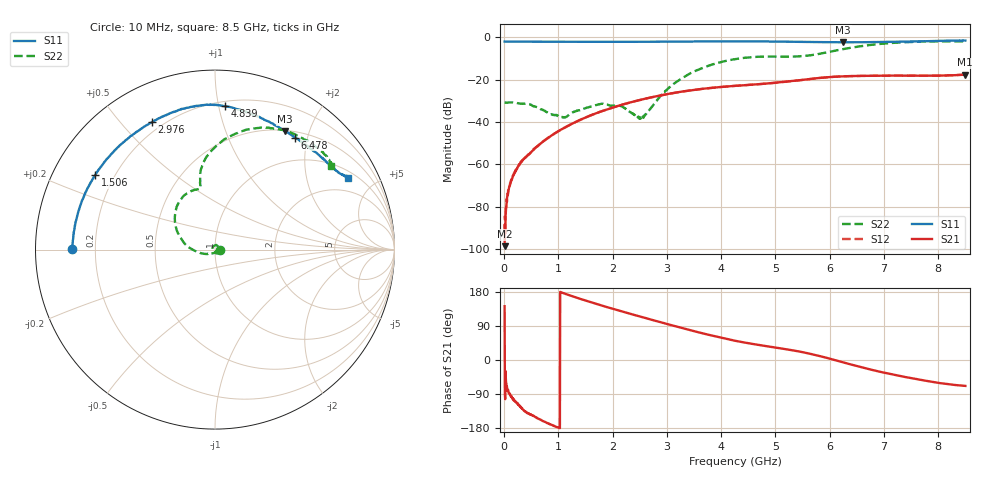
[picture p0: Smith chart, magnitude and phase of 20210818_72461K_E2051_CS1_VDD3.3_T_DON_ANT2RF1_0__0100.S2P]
!Agilent Technologies,E5071C,MY46417908,A.11.23
!Date: Wed Aug 18 14:23:03 2021
!Data & Calibration Information:
!Freq	S11:SOLT2(ON)	S21:SOLT2(ON)	S12:SOLT2(ON)	S22:SOLT2(ON)
!PortZ  Port1:50+j0  Port2:50+j0
!Above PortZ is port z conversion or system Z0 setting when saving the data.
!When reading, reference impedance value at option line is always used.
# Hz S dB R 50
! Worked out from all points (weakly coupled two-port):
!   1601 points, 10 MHz to 8.5 GHz, reference 50 ohm
!   highest |S21| = -17.62 dB at 8.495 GHz (marker M1); lowest = -98.6 dB at 10 MHz (marker M2)
!   lowest |S11| = -2.3 dB at 6.25 GHz (marker M3), VSWR 7.51, Z = 25.6 + j81.4 ohm
!   |S11| at or under -10 dB: nowhere
!   |S22| runs from -38.4 to -1.8 dB; largest |S21 - S12| = 0.00061
!   S11 on the Smith chart (normalised r, x): 10 MHz: 0.11, +0.00; 1.506 GHz: 0.13, +0.28; 2.976 GHz: 0.16, +0.61; 4.839 GHz: 0.23, +1.04; 6.478 GHz: 0.59, +1.79; 8.5 GHz: 1.27, +3.52
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1e7  -1.96 179.7  -98.60 141.9  -92.20 -89.4  -30.66 -2.2
1.532688e8  -2.01 176.8  -66.42 -101.8  -65.96 -100.6  -30.70 -12.6
3.496e8  -2.02 172.7  -57.69 -130.4  -57.79 -130.0  -31.35 -35.5
7.051188e8  -2.04 165.0  -49.39 -160.3  -49.40 -160.4  -34.19 -81.0
1.097781e9  -2.07 156.8  -42.89 176.0  -42.84 176.3  -37.78 -171.1
1.426769e9  -2.08 149.8  -38.67 160.2  -38.67 160.2  -34.09 120.5
1.506362e9  -2.09 148.1  -37.78 156.8  -37.80 156.7  -33.33 107.5
1.7929e9  -2.10 141.8  -34.93 143.9  -34.93 144.0  -31.35 75.0
2.116581e9  -2.10 134.6  -32.24 130.5  -32.25 130.4  -32.17 35.4
2.530469e9  -2.08 125.7  -29.39 113.8  -29.39 113.7  -37.70 -55.7
2.843538e9  -2.04 119.0  -27.61 101.3  -27.61 101.2  -28.80 -140.5
2.976194e9  -2.02 116.3  -26.96 96.1  -26.95 96.1  -25.29 -154.2
3.4909e9  -1.93 106.8  -24.82 76.5  -24.82 76.5  -16.20 173.3
4.255e9  -1.86 94.6  -22.89 50.9  -22.90 50.9  -10.28 135.7
4.838688e9  -1.93 86.1  -21.78 36.4  -21.78 36.4  -9.09 113.2
5.671769e9  -2.17 71.7  -19.55 15.5  -19.55 15.6  -8.37 102.6
6.25015e9  -2.33 59.6  -18.40 -6.4  -18.42 -6.4  -5.55 94.2
6.478319e9  -2.32 54.6  -18.24 -15.2  -18.26 -15.2  -4.53 87.6
7.088538e9  -2.12 42.1  -18.07 -35.9  -18.10 -36.1  -2.73 68.5
7.921619e9  -1.70 30.6  -18.09 -58.3  -18.08 -58.3  -1.88 44.5
8.494694e9  -1.47 28.4  -17.62 -68.3  -17.64 -68.6  -1.96 35.7
8.5e9  -1.48 28.4  -17.62 -68.3  -17.64 -68.6  -1.98 35.6
